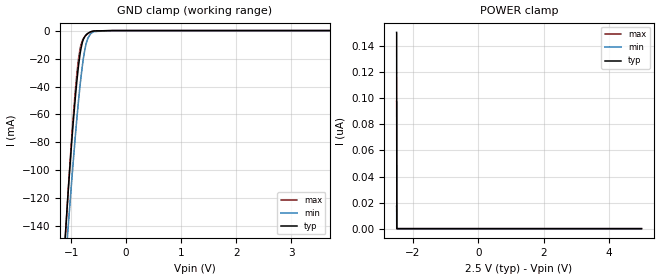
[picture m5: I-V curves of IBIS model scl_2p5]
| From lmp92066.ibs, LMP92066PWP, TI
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|   scl_2p5 Model
[Model]   scl_2p5
Model_type   Input
Vinl = 0.75
Vinh = 1.75
|   typ   min   max
|   (nom PVT)   (fast PVT)   (slow PVT)
C_comp   3.837e-13   3.592e-13   4.249e-13
[Model spec]
|subparameter
Vinl   0.75   0.675   0.825
Vinh   1.75   1.575   1.925
| Where nom  PVT is Nominal Process, 2.5V, 25C
|   Fast PVT is Strong Process,  2.75V, -25C
|   Slow PVT is Weak Process,   2.25V, 125C
[Voltage Range]   2.5   2.25   2.75
|Junction Temperature
[Temperature Range]   25   125   -25
[Power Clamp Reference]   2.5   2.25   2.75
[GND Clamp Reference]   0   0   0
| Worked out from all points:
|   GND clamp passes 1 mA (typ) near -0.65 V on its own axis
[GND Clamp]
|   Voltage   I(typ)   I(min)   I(max)
-2.5V     -1.154A    -1.002A    -1.199A
-1.103V   -144.6mA   -166.2mA   -146.3mA
-1.062V   -120.2mA   -144.7mA   -120.1mA
-965.5mV  -67.34mA   -95.46mA   -63.1mA
-917.5mV  -45.04mA   -72.52mA   -39.64mA
-866.5mV  -25.36mA   -50.39mA   -20.3mA
-797.7mV  -8.723mA   -25.71mA   -7.295mA
-747.2mV  -3.967mA   -12.93mA   -4.082mA
-697.7mV  -1.983mA   -5.664mA   -2.226mA
-648.2mV  -922.4uA   -2.353mA   -1.021mA
-250mV    0A         0A         0A
5V        0A         0A         0A
[POWER Clamp]
|   Voltage   I(typ)   I(min)   I(max)
-2.5V     150.6nA    17.41nA    97.71nA
-2.498V   150.2nA    12.88nA    97.46nA
-2.498V   150.2nA    12.16nA    97.43nA
-2.497V   142.7nA    11.45nA    97.4nA
-2.495V   90.1nA     0A         66.41nA
-2.495V   75.08nA    0A         57.56nA
-2.494V   60.06nA    0A         48.7nA
-2.493V   22.52nA    0A         26.56nA
-2.493V   0A         0A         13.28nA
-2.492V   0A         0A         0A
5V        0A         0A         0A
